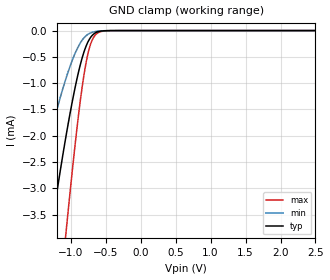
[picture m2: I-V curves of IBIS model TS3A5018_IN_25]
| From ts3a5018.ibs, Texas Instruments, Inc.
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[Model]   TS3A5018_IN_25
Model_type  Input
Vinl=0.7
Vinh=1.7
| variable   typ   min   max
C_comp   2.35pF   1.58pF   2.79pF
[Temperature Range]   40   100   -40
| Ambient temperature   25   85   -40
[Voltage range]   2.5   2.3   2.7
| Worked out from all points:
|   GND clamp passes 1 mA (typ) near -0.93 V on its own axis
[GND Clamp]
| TS3A5018_IN_25
|   Voltage   I(typ)   I(min)   I(max)
-2.5V     -18.36mA   -11.41mA   -27.99mA
-1.595V   -6.977mA   -3.857mA   -11.79mA
-1.305V   -4.021mA   -2.053mA   -7.198mA
-1.275V   -3.743mA   -1.89mA    -6.75mA
-1.065V   -1.972mA   -889.7uA   -3.78mA
-960mV    -1.217mA   -498.4uA   -2.421mA
-870mV    -676.3uA   -247uA     -1.386mA
-800mV    -358.8uA   -120.3uA   -741.2uA
-745mV    -188.6uA   -62.27uA   -380.7uA
-660mV    -52.49uA   -21.34uA   -100.1uA
-515mV    -3.473uA   -2.323uA   -7.329uA
2.5V      154.1pA    8.876pA    1.606nA
